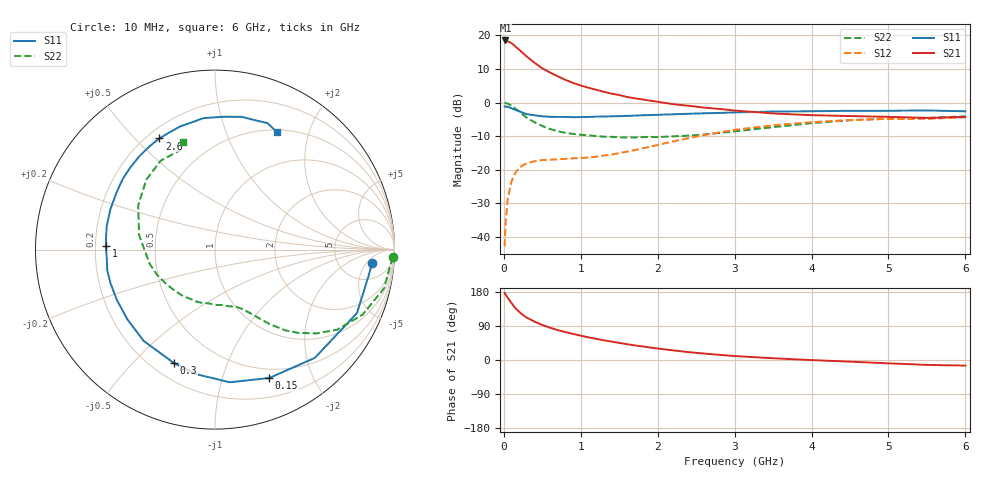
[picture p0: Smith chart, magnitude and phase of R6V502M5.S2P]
! SIEMENS Small Signal Semiconductors
! BFR193
! Si NPN RF Bipolar Junction Transistor in SOT23
! VCE = 0.5 V  IC = 2.5 mA
! Common Emitter S-Parameters:  May  1996
# GHz  S  MA  R  50
!  f  S11  S21  S12  S22
! GHz  MAG  ANG  MAG  ANG  MAG  ANG  MAG  ANG
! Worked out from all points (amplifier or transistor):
!   36 points, 10 MHz to 6 GHz, reference 50 ohm
!   highest |S21| = 18.5 dB at 20 MHz (marker M1)
!   |S21| within 3 dB of that: start of sweep to 211.2 MHz
!   unconditionally stable (mu >= 1): 1.038 GHz to 2.432 GHz; 5.025 GHz to end of sweep
!   at 250 MHz: K = 0.28, MSG = 16.6 dB, |S12| = -18.6 dB
!   at 1.4 GHz: K = 1.14, MAG = 6.8 dB, |S12| = -15.5 dB
!   at 6 GHz: K = 1.01, MAG = -0.6 dB, |S12| = -4.4 dB
!   S11 on the Smith chart (normalised r, x): 10 MHz: 11, -7; 150 MHz: 0.40, -1.43; 300 MHz: 0.29, -0.66; 1 GHz: 0.24, +0.01; 2.6 GHz: 0.25, +0.59; 6 GHz: 0.52, +1.52
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0.01  0.8781 -5.0  8.373 177.2  0.0073 87.7  0.9928 -2.5
0.02  0.8677 -10.0  8.393 173.6  0.0145 86.1  0.9808 -5.1
0.05  0.8663 -24.1  8.163 164.4  0.0365 76.5  0.967 -12.8
0.1  0.8207 -47.3  7.641 150.0  0.0674 65.0  0.8986 -23.8
0.15  0.7767 -67.1  6.826 137.0  0.0902 55.1  0.8132 -33.3
0.2  0.7438 -83.7  6.099 127.1  0.1063 48.2  0.7327 -39.6
0.25  0.7014 -98.8  5.426 118.2  0.1176 42.6  0.6564 -45.0
0.3  0.6718 -110.0  4.822 111.5  0.1246 38.4  0.5943 -49.1
0.4  0.6456 -128.0  3.896 101.2  0.1344 33.1  0.5082 -54.1
0.5  0.6241 -141.4  3.236 92.5  0.1393 30.2  0.4478 -57.7
0.6  0.6146 -152.8  2.798 85.2  0.1414 29.0  0.4035 -61.1
0.7  0.6116 -162.0  2.461 79.0  0.1429 28.8  0.375 -64.1
0.8  0.6115 -169.0  2.176 73.7  0.1453 29.3  0.3538 -66.9
1  0.6084 178.3  1.794 64.1  0.1493 31.6  0.3324 -72.5
1.1  0.6113 172.9  1.664 59.8  0.1525 33.4  0.3252 -76.2
1.6  0.6333 150.5  1.212 41.6  0.1861 43.7  0.3025 -96.3
2.2  0.6685 129.4  0.946 25.4  0.2637 47.5  0.3144 -124.6
2.6  0.6925 116.6  0.841 17.1  0.328 44.6  0.3345 -146.2
3.5  0.7355 94.9  0.688 4.6  0.4591 30.1  0.4303 169.3
4.5  0.7543 78.7  0.63 -4.4  0.5491 12.8  0.5458 134.5
5.5  0.7632 67.5  0.591 -12.9  0.573 -2.7  0.5882 108.4
6  0.7408 62.4  0.611 -14.8  0.6034 -7.2  0.6246 106.7
